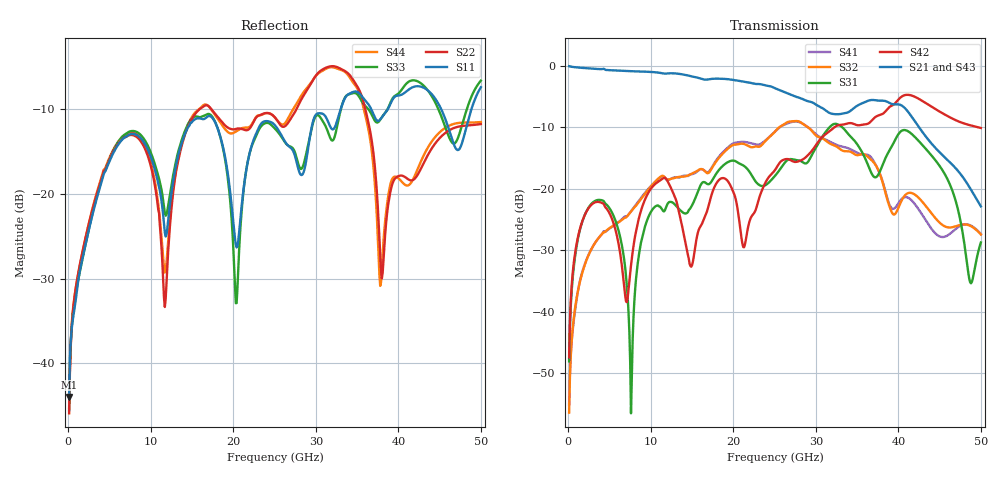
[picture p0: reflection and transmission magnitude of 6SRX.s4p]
! DAC39RF10ACK
! 256-pin FCBGA package
! Texas Instruments 8/20/2022
! Single-ended  S-parameters
! PORT#  PORT_NAME  NET_NAME
! PORT1:  xSRXN.DIEBUMP  xSRXN
! PORT2:  xSRXN.BGA  xSRXN
! PORT3:  xSRXP.DIEBUMP  xSRXP
! PORT4:  xSRXP.BGA  xSRXP
! Touchstone Ver. 1.0
! Number of ports is 4
# Hz	S	MA	R	50.000000
! SCATTERING PARAMETERS  :
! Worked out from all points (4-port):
!   500 points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, 100 MHz to 50 GHz, reference 50 ohm
!   strongest paths, dB at 100 MHz, 12.6 GHz, 25.1 GHz, 37.6 GHz, 50 GHz:
!     S21: 0.0, -1.2, -3.7, -5.7, -22.9
!     S43: 0.0, -1.2, -3.7, -5.5, -23.0
!     S42: -47.4, -20.3, -16.9, -8.1, -10.1
!     S31: -48.1, -22.2, -17.8, -17.6, -28.8
!     S32: -56.5, -18.3, -10.6, -17.0, -27.5
!     S41: -55.1, -18.3, -10.6, -17.1, -27.4
!   lowest |S11| = -44.0 dB at 100 MHz (marker M1), VSWR 1.01, Z = 50.5 + j0.422 ohm
!   |S11| at or under -10 dB: start of sweep to 33 GHz; 36.72 GHz to 38.71 GHz (1.993 GHz wide, 5.28 % of centre); 45.2 GHz to 48.85 GHz (3.643 GHz wide, 7.75 % of centre)
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1e8  0.006302 41.5  0.9958 -2.6  0.003818 84.3  0.001537 -100.3
     0.9946 -2.7  0.005047 38.1  0.001572 -100.0  0.004412 83.3
     0.00393 82.8  0.001503 -99.9  0.005256 40.2  0.9955 -2.7
     0.00175 -103.7  0.004242 83.9  0.9956 -2.7  0.005432 39.8
3.8e9  0.108 12.9  0.9423 -91.0  0.08092 -7.5  0.04079 166.2
       0.9415 -91.0  0.1133 -31.1  0.04054 165.5  0.07787 0.1
       0.0811 -7.8  0.04071 165.2  0.1111 11.1  0.9448 -91.9
       0.0406 165.9  0.07782 0.1  0.9422 -91.6  0.1156 -30.5
7.4e9  0.2243 -64.2  0.9064 -175.3  0.006971 -88.0  0.06282 91.7
       0.9044 -175.3  0.2226 -107.9  0.06286 91.0  0.01682 153.7
       0.006845 -86.5  0.06264 90.7  0.2336 -66.1  0.9006 -176.7
       0.06286 92.5  0.01757 154.8  0.9033 -176.6  0.2307 -108.6
1.47e10  0.2547 -86.7  0.827 11.0  0.06756 168.8  0.1295 -86.0
         0.8288 10.8  0.2621 -75.8  0.1288 -88.7  0.02529 20.6
         0.06807 167.2  0.1297 -88.1  0.2682 -91.6  0.8273 8.5
         0.1305 -86.4  0.02447 11.9  0.826 8.7  0.2697 -75.0
2.23e10  0.1986 -48.6  0.7213 -168.2  0.1266 -142.0  0.2348 86.0
         0.7213 -168.5  0.2579 -122.5  0.2203 83.9  0.06465 50.9
         0.1264 -142.6  0.2175 84.3  0.1956 -63.1  0.716 -171.8
         0.2332 85.7  0.06074 49.3  0.7112 -171.9  0.2612 -122.1
2.96e10  0.2621 -71.3  0.5007 17.9  0.1907 -159.3  0.2923 -124.5
         0.5029 18.0  0.4663 -133.8  0.2915 -129.5  0.207 177.0
         0.1928 -159.9  0.2914 -130.1  0.2567 -82.4  0.4827 14.7
         0.294 -124.2  0.2068 176.8  0.4848 15.2  0.4689 -136.9
5e10  0.4277 -89.7  0.08567 -74.3  0.0271 -157.5  0.04397 176.0
      0.0717 -76.3  0.2589 -138.8  0.04383 -174.9  0.2949 -26.7
      0.0365 -155.8  0.0424 164.7  0.4676 -99.5  0.07583 -76.0
      0.04276 -167.5  0.3121 -28.0  0.07096 -83.5  0.2661 -141.0
